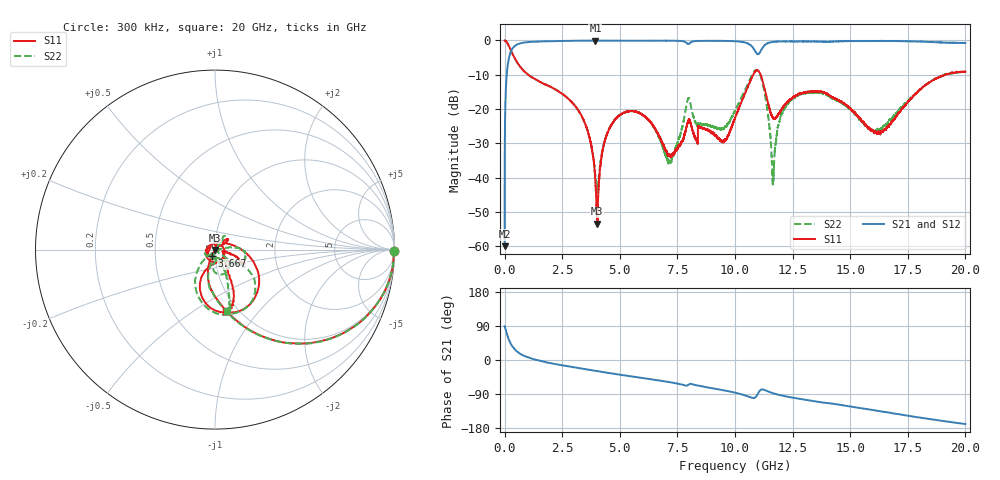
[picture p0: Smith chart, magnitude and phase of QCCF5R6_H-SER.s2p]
!{QCCF5R6}
!Johanson Technology Inc.
!www.johansontechnology.com
!Test Board Conditions:
!Substrate Type  RO4350B
!Substrate Thickness  10 mil
!Substrate Dk  3.66
!TL Type: GCPW
!TL Trace Width  21 mil
!TL Gap  20 mil
!Electrode orientation  Horizontal
!DUT TOPOLOGY	SERIES
!Mounting Pad LxW  16x21 mil
! Created Sat Jan  9 18:15:19 2021
# hz S ma R 50
! 2 Port Network Data from SP1.SP block
! freq  magS11  angS11  magS21  angS21  magS12  angS12  magS22  angS22
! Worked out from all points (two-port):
!   20001 points, 300 kHz to 20 GHz, reference 50 ohm
!   highest |S21| = -0.03 dB at 3.94 GHz (marker M1); lowest = -60.0 dB at 300 kHz (marker M2)
!   |S21| within 3 dB of the highest: 284.5 MHz to 10.87 GHz (10.58 GHz wide, 190 % of centre); 11.12 GHz to end of sweep
!   lowest |S11| = -53.5 dB at 4.019 GHz (marker M3), VSWR 1.00, Z = 50.2 - j0.134 ohm
!   |S11| at or under -10 dB: 1.031 GHz to 10.79 GHz (9.761 GHz wide, 165 % of centre); 11.11 GHz to 19.13 GHz (8.012 GHz wide, 53 % of centre); 19.12669 GHz to 19.13385 GHz (7.16 MHz wide, 0.0374 % of centre)
!   |S22| runs from -44.6 to 0.0 dB; largest |S21 - S12| = 0.016
!   S11 on the Smith chart (normalised r, x): 300 kHz: open; 3.667 GHz: 0.96, -0.07; 20 GHz: 0.88, -0.69
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300000  0.9957 -0.4  0.001001 89.2  0.0009993 86.5  0.9955 -0.5
1.133e8  0.9245 -23.5  0.3774 66.2  0.3772 66.3  0.9243 -23.5
3.293e8  0.6513 -52.8  0.7521 36.6  0.7519 36.7  0.6512 -52.9
1.0203e9  0.3184 -82.6  0.9455 6.8  0.946 6.9  0.317 -83.5
3.3343e9  0.08038 -113.4  0.992 -22.5  0.9929 -22.5  0.08005 -106.2
3.6673e9  0.04048 -116.1  0.9946 -25.9  0.9944 -25.8  0.04015 -103.3
3.9403e9  0.008695 -107.8  0.9962 -28.5  0.9951 -28.5  0.01017 -76.3
4.0193e9  0.002122 -38.9  0.9951 -29.4  0.9951 -29.3  0.006389 -19.8
4.3283e9  0.03232 47.3  0.9939 -32.4  0.9941 -32.4  0.03265 53.5
4.8663e9  0.07485 44.2  0.9917 -37.5  0.992 -37.5  0.0747 57.1
6.6673e9  0.04289 35.0  0.9919 -53.8  0.9921 -53.7  0.04174 47.4
7.1663e9  0.02183 71.9  0.9903 -58.6  0.9897 -58.5  0.01744 -9.2
7.9723e9  0.06739 -66.2  0.8891 -65.5  0.8886 -65.5  0.1432 -66.1
9.4543e9  0.03376 113.4  0.985 -79.4  0.9835 -79.4  0.05184 -91.5
1.00003e10  0.07333 27.7  0.9732 -86.2  0.9728 -86.2  0.09338 -40.5
1.10153e10  0.3596 -78.8  0.6333 -86.8  0.6327 -87.0  0.3601 -86.1
1.13403e10  0.1647 -116.4  0.8806 -80.5  0.8801 -80.5  0.1331 -132.1
1.16623e10  0.07322 -82.9  0.9544 -87.9  0.9534 -87.9  0.01025 -47.4
1.21663e10  0.1151 -35.0  0.9689 -95.5  0.969 -95.5  0.1029 6.8
1.33343e10  0.1792 -25.9  0.9659 -107.7  0.9671 -107.6  0.1742 -12.5
1.66673e10  0.0554 -29.8  0.9832 -138.6  0.9773 -139.0  0.06629 -77.2
2e10  0.3494 -79.8  0.9197 -169.1  0.9099 -168.9  0.3485 -78.7
